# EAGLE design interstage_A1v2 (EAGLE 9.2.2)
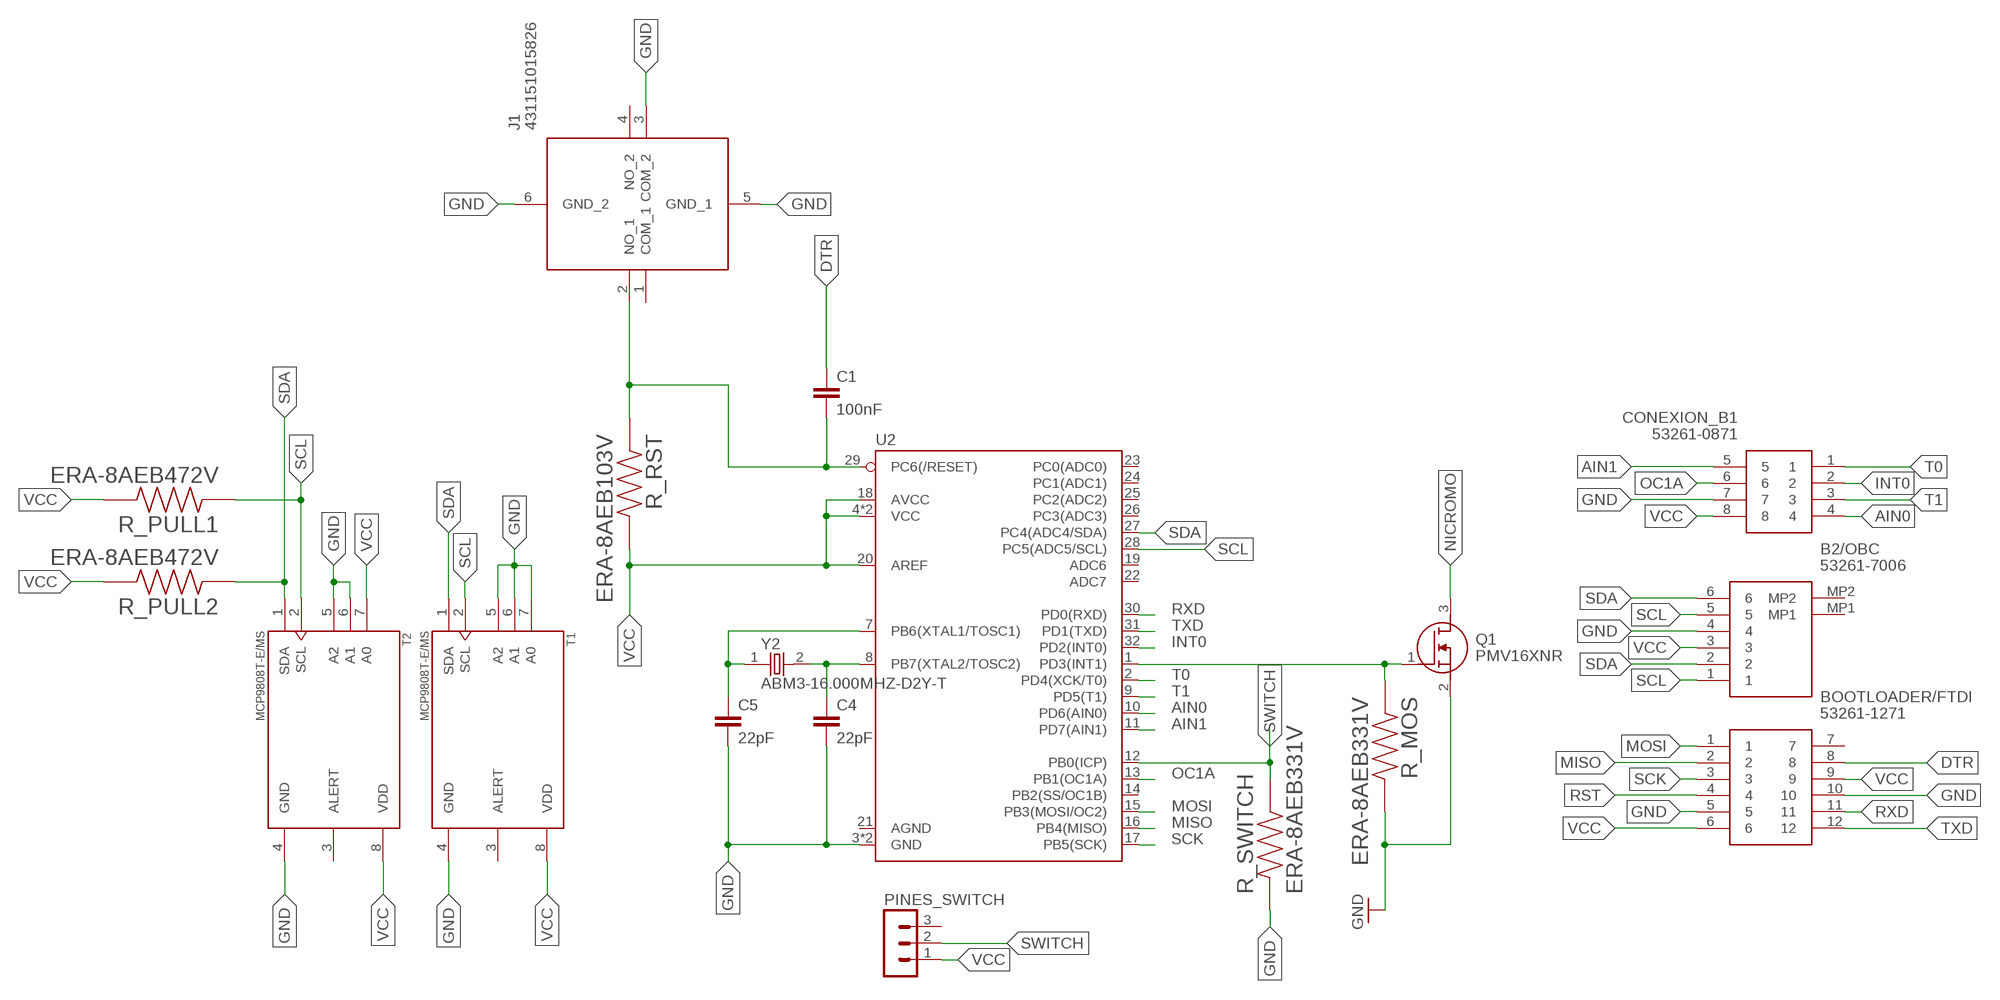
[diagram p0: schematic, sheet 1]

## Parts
B2/OBC  53261-7006  [532617006]
BOOTLOADER/FTDI  53261-1271  [53261-1271]
C1  100nF  C-EUC0805K  [C0805K]
C4  22pF  C-EUC0603K  [C0603K]
C5  22pF  C-EUC0603K  [C0603K]
CONEXION_B1  53261-0871  [53261-0871]
J1  431151015826  [431151015826]
PINES_SWITCH  MA03-1  [MA03-1]
Q1  PMV16XNR  [SOT95P230X110-3N]
R_MOS  ERA-8AEB331V  [RESC3216X70N]
R_PULL1  ERA-8AEB472V  [RESC3216X70N]
R_PULL2  ERA-8AEB472V  [RESC3216X70N]
R_RST  ERA-8AEB103V  [RESC3216X70N]
R_SWITCH  ERA-8AEB331V  [RESC3216X70N]
T1  MCP9808T-E/MS  [SOP65P490X110-8N]
T2  MCP9808T-E/MS  [SOP65P490X110-8N]
U2  ATMEGA328P_TQFP  [TQFP32-08]
Y2  ABM3-16.000MHZ-D2Y-T  [XTAL500X320X130N]

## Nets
AIN0: CONEXION_B1.4 U2.10(PD6(AIN0))
AIN1: CONEXION_B1.5 U2.11(PD7(AIN1))
DTR: BOOTLOADER/FTDI.8 C1.1
GND: B2/OBC.4 BOOTLOADER/FTDI.5 BOOTLOADER/FTDI.10 C4.2 C5.2 CONEXION_B1.7 J1.3(COM_2) J1.5(GND_1) J1.6(GND_2) Q1.2(S) R_MOS.2 R_SWITCH.1 T1.4(GND) T1.5(A2) T1.6(A1) T1.7(A0) T2.4(GND) T2.5(A2) T2.6(A1) U2.3(GND) U2.5(GND)
INT0: CONEXION_B1.2 U2.32(PD2(INT0))
INT1: Q1.1(G) R_MOS.1 U2.1(PD3(INT1))
MISO: BOOTLOADER/FTDI.2 U2.16(PB4(MISO))
MOSI: BOOTLOADER/FTDI.1 U2.15(PB3(MOSI/OC2))
N$1: C5.1 U2.7(PB6(XTAL1/TOSC1)) Y2.1
N$2: C4.1 U2.8(PB7(XTAL2/TOSC2)) Y2.2
NICROMO: Q1.3(D)
OC1A: CONEXION_B1.6 U2.13(PB1(OC1A))
RST: BOOTLOADER/FTDI.4 C1.2 J1.2(NO_1) R_RST.1 U2.29(PC6(/RESET))
RXD: BOOTLOADER/FTDI.11 U2.30(PD0(RXD))
SCK: BOOTLOADER/FTDI.3 U2.17(PB5(SCK))
SCL: B2/OBC.1 B2/OBC.5 R_PULL1.1 T1.2(SCL) T2.2(SCL) U2.28(PC5(ADC5/SCL))
SDA: B2/OBC.2 B2/OBC.6 R_PULL2.1 T1.1(SDA) T2.1(SDA) U2.27(PC4(ADC4/SDA))
SWITCH: PINES_SWITCH.2 R_SWITCH.2 U2.12(PB0(ICP))
T0: CONEXION_B1.1 U2.2(PD4(XCK/T0))
T1: CONEXION_B1.3 U2.9(PD5(T1))
TXD: BOOTLOADER/FTDI.12 U2.31(PD1(TXD))
VCC: B2/OBC.3 BOOTLOADER/FTDI.6 BOOTLOADER/FTDI.9 CONEXION_B1.8 PINES_SWITCH.1 R_PULL1.2 R_PULL2.2 R_RST.2 T1.8(VDD) T2.7(A0) T2.8(VDD) U2.4(VCC) U2.6(VCC) U2.18(AVCC) U2.20(AREF)
Unconnected: B2/OBC.MP1 B2/OBC.MP2 BOOTLOADER/FTDI.7 J1.1(COM_1) J1.4(NO_2) PINES_SWITCH.3 T1.3(ALERT) T2.3(ALERT) U2.14(PB2(SS/OC1B)) U2.19(ADC6) U2.21(AGND) U2.22(ADC7) U2.23(PC0(ADC0)) U2.24(PC1(ADC1)) U2.25(PC2(ADC2)) U2.26(PC3(ADC3))

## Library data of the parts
B2/OBC = SamacSys_Parts:53261-7006: 1.25mm Pitch, PicoBlade PCB Header, Single Row, Right-Angle, Surface Mount, Gold (Au) Plating, Friction Lock, Circuits, Tape and Reel Source: Datasheet; DESCRIPTION: 1.25mm Pitch, PicoBlade PCB Header, Single Row, Right-Angle, Surface Mount, Gold (Au) Plating, Friction Lock, Circuits, Tape and Reel; HEIGHT: 3.6mm; MANUFACTURER_NAME: Molex; MANUFACTURER_PART_NUMBER: 53261-7006; MOUSER_PART_NUMBER: 538-53261-7006; MOUSER_PRICE-STOCK: https://www.mouser.co.uk/ProductDetail/Molex/53261-7006?qs=0lSvoLzn4L%2FSBef0BTU2GA%3D%3D
BOOTLOADER/FTDI = SamacSys_Parts:53261-1271: Molex PICOBLADE Series, Series Number 53261, 1.25mm Pitch 12 Way 1 Row Right Angle PCB Header, Solder Termination, 1A Source: Datasheet; DESCRIPTION: Molex PICOBLADE Series, Series Number 53261, 1.25mm Pitch 12 Way 1 Row Right Angle PCB Header, Solder Termination, 1A; HEIGHT: mm; MANUFACTURER_NAME: Molex; MANUFACTURER_PART_NUMBER: 53261-1271; MOUSER_PART_NUMBER: 538-53261-1271; MOUSER_PRICE-STOCK: https://www.mouser.co.uk/ProductDetail/Molex/53261-1271?qs=%252B72YyncTwW8ciqCjtXK7Ww%3D%3D
C1 C4 C5 = rcl:C-EU: CAPACITOR, European symbol; SPICEPREFIX: C
CONEXION_B1 = SamacSys_Parts:53261-0871: Molex PICOBLADE Series, Series Number 53261, 1.25mm Pitch, 8 Way 1 Row Shrouded Right Angle PCB Header, Surface Mount Source: Datasheet; DESCRIPTION: Molex PICOBLADE Series, Series Number 53261, 1.25mm Pitch, 8 Way 1 Row Shrouded Right Angle PCB Header, Surface Mount; HEIGHT: mm; MANUFACTURER_NAME: Molex; MANUFACTURER_PART_NUMBER: 53261-0871; MOUSER_PART_NUMBER: 538-53261-0871; MOUSER_PRICE-STOCK: https://www.mouser.co.uk/ProductDetail/Molex/53261-0871?qs=%252B72YyncTwW%252BggfdCJ7Netw%3D%3D
J1 = SamacSys_Parts:431151015826: White Tactile Tactile Switch, NO 20 mA 0.3mm Surface Mount Source: Datasheet; DESCRIPTION: White Tactile Tactile Switch, NO 20 mA 0.3mm Surface Mount; HEIGHT: 1.6mm; MANUFACTURER_NAME: Wurth Elektronik; MANUFACTURER_PART_NUMBER: 431151015826; MOUSER_PART_NUMBER: 710-431151015826; MOUSER_PRICE-STOCK: https://www.mouser.co.uk/ProductDetail/Wurth-Elektronik/431151015826?qs=wr8lucFkNMWt0fEnpc%252BesA%3D%3D
PINES_SWITCH = con-lstb:MA03-1: PIN HEADER; OC_FARNELL: unknown; OC_NEWARK: unknown
Q1 = SamacSys_Parts:PMV16XNR: Nexperia PMV16XNR N-channel MOSFET, 8.6 A, 20 V PMV16XN, 3-Pin SOT-23 Source: Datasheet; DESCRIPTION: Nexperia PMV16XNR N-channel MOSFET, 8.6 A, 20 V PMV16XN, 3-Pin SOT-23; HEIGHT: 1.1mm; MANUFACTURER_NAME: Nexperia; MANUFACTURER_PART_NUMBER: PMV16XNR; MOUSER_PART_NUMBER: 771-PMV16XNR; MOUSER_PRICE-STOCK: https://www.mouser.com/Search/Refine.aspx?Keyword=771-PMV16XNR
R_MOS R_SWITCH = resistor_330_smd:ERA-8AEB331V; DESCRIPTION: 330 Ohms ±0.1% 0.25W, 1/4W Chip Resistor 1206 (3216 Metric) Automotive AEC-Q200 Thin Film; DIGI-KEY_PART_NUMBER: P330BCCT-ND; MF: Panasonic Electronic; MP: ERA-8AEB331V; PACKAGE: 3216 Panasonic Electronic Components
R_PULL1 R_PULL2 = resistor_4700_smd:ERA-8AEB472V; DESCRIPTION: RES SMD 4.7K OHM 0.1% 1/4W 1206; DIGI-KEY_PART_NUMBER: P4.7KBCCT-ND; DIGIKEY-PURCHASE-URL: https://snapeda.com/shop?store=DigiKey&id=3718815; MF: Panasonic; MP: ERA-8AEB472V; PACKAGE: 3216 Panasonic Electronic Components
R_RST = resistor_10000_smd:ERA-8AEB103V; DESCRIPTION: 10 kOhms ±0.1% 0.25W, 1/4W Chip Resistor 1206 (3216 Metric) Automotive AEC-Q200 Thin Film; DIGI-KEY_PART_NUMBER: P10KBCCT-ND; DIGIKEY-PURCHASE-URL: https://snapeda.com/shop?store=DigiKey&id=3229630; MF: Panasonic Electronic Components; MP: ERA-8AEB103V; PACKAGE: 3216 Panasonic Electronic Components
T1 T2 = sensorSPEL:MCP9808T-E/MS: Board Mount Temperature Sensors Silicon temp sensor with I2C interface; DESCRIPTION: Temperature Sensor Digital, Local -40°C ~ 125°C 10 b 8-MSOP; DIGI-KEY_PART_NUMBER: MCP9808T-E/MSCT-ND; MF: Microchip; MP: MCP9808T-E/MS; PACKAGE: MSOP-8 Microchip
U2 = SparkFun-IC-Microcontroller:ATMEGA328P_TQFP: Popular 328P in QFP Storefront component: ATmega328 - TQFP (COM-13448) Datasheet SparkFun Products SparkFun RedBoard - Programmed with Arduino (DEV-12757) Arduino Pro Mini 328 - 5V/16MHz (DEV-11113) Arduino Pro Mini 328 - 3.3V/8MHz (DEV-11114) SparkFun OpenLog (DEV-13712) SparkFun MicroView - OLED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; PROD_ID: IC-09069
Y2 = ABM3-16.000MHZ-D2Y-T:ABM3-16.000MHZ-D2Y-T: Crystals 12MHz 18pF 30ppm -40C +85C; DESCRIPTION: 16MHz ±20ppm Crystal 18pF 40 Ohms 2-SMD, No Lead; DIGI-KEY_PART_NUMBER: 535-10638-1-ND; DIGIKEY-PURCHASE-URL: https://snapeda.com/shop?store=DigiKey&id=55267; MF: Abracon; MP: ABM3-16.000MHZ-D2Y-T; PACKAGE: SMD-2 Abracon

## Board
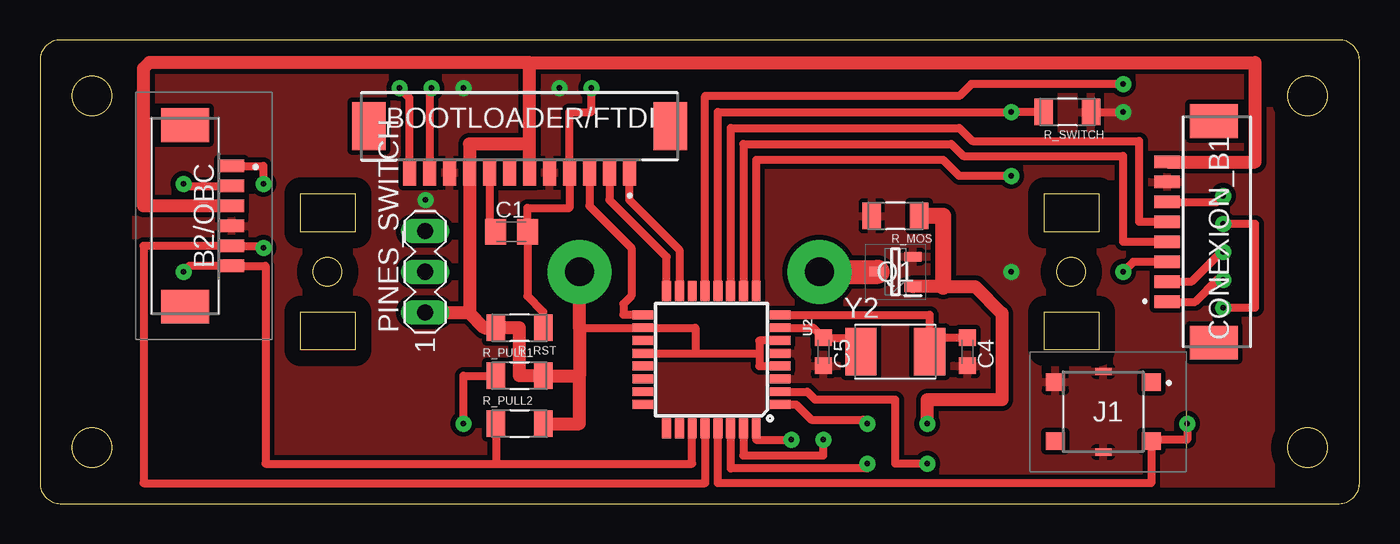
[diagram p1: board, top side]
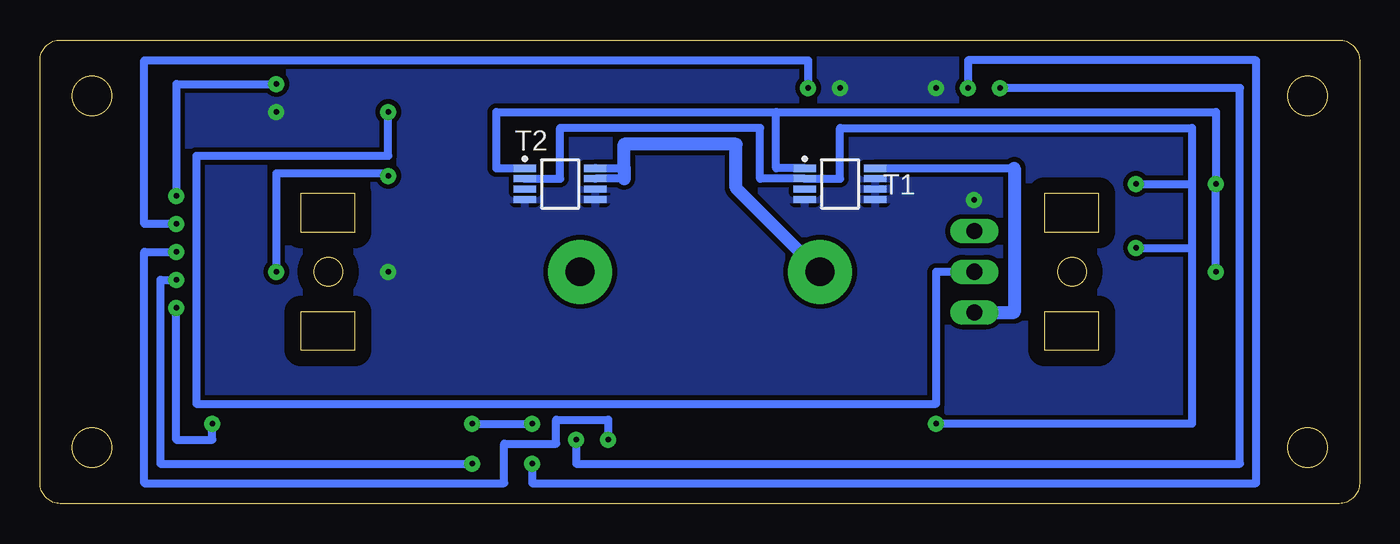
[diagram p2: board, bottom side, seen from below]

Size 82.5 x 29 mm. Coordinates in mm from the lower left corner, seen from the top.
Outline: 16.3,17 16.3,19.4 19.7,19.4 19.7,17 16.3,17
Outline: 62.8,9.6 62.8,12 66.2,12 66.2,9.6 62.8,9.6
Outline: 16.3,9.6 16.3,12 19.7,12 19.7,9.6 16.3,9.6
Outline: 62.8,17 62.8,19.4 66.2,19.4 66.2,17 62.8,17
Outline: 0,1.27 arc90 1.27,0 81.23,0 arc90 82.5,1.27 82.5,27.73 arc90 81.23,29 1.27,29 arc90 0,27.73 0,1.27
Outline: circle at 3.25,25.5 radius 1.25
Outline: circle at 79.25,3.5 radius 1.25
Outline: circle at 79.25,25.5 radius 1.25
Outline: circle at 3.25,3.5 radius 1.25
Outline: circle at 17.98,14.5 radius 0.9
Outline: circle at 64.48,14.5 radius 0.9
Copper layers (1*16): Top 0.035mm / dielectric 1.5mm / Bottom 0.035mm
Design rules "default *": minimum track width 6mil, minimum drill 0.35mm, track to track 0.3mm, track to pad 6mil, pad to pad 6mil, via to via 6mil, smd to smd 6mil, copper to edge 40mil, drill to drill 6mil, minimum pad ring 10mil, minimum via ring 8mil, stop-mask expansion 4mil, vias tented up to drill 0mil, thermal gap 10mil

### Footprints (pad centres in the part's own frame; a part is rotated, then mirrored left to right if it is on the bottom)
532617006 = smd 0.8 x 1.6: 1 3.125,-2.5; 2 1.875,-2.5; 3 0.625,-2.5; 4 -0.625,-2.5; 5 -1.875,-2.5; 6 -3.125,-2.5 | smd 2.1 x 3: MP1 5.675,0.4; MP2 -5.675,0.4
53261-1271 = smd 0.8 x 1.6: 1 -6.875,0.8; 2 -5.625,0.8; 3 -4.375,0.8; 4 -3.125,0.8; 5 -1.875,0.8; 6 -0.625,0.8; 7 0.625,0.8; 8 1.875,0.8; 9 3.125,0.8; 10 4.375,0.8; 11 5.625,0.8; 12 6.875,0.8 | smd 2.1 x 3: 13 -9.425,-2.1; 14 9.425,-2.1
C0805K = smd 1.3 x 1.6: 1 -1,0; 2 1,0
C0603K = smd 1.05 x 1.08: 1 -0.875,0; 2 0.875,0
53261-0871 = smd 0.8 x 1.6: 1 -4.375,1.004; 2 -3.125,1.004; 3 -1.875,1.004; 4 -0.625,1.004; 5 0.625,1.004; 6 1.875,1.004; 7 3.125,1.004; 8 4.375,1.004 | smd 2.1 x 3: 9 6.925,-1.896; 10 -6.925,-1.896
431151015826 = smd 1.2 x 1.1: 1 -3,-1.85; 2 -3,1.85; 3 3,-1.85; 4 3,1.85 | smd 1 x 0.45: 5 0,-2.525; 6 0,2.525
MA03-1 = drill 1.016 long: 1 -2.54,0; 2 0,0; 3 2.54,0
SOT95P230X110-3N = smd 1.05 x 0.6: 1 -1.1,0.95; 2 -1.1,-0.95; 3 1.1,0
RESC3216X70N = smd 1.16 x 1.68: 1 -1.475,0; 2 1.475,0
SOP65P490X110-8N = smd 1.4 x 0.45: 1 -2.2,0.975; 2 -2.2,0.325; 3 -2.2,-0.325; 4 -2.2,-0.975; 5 2.2,-0.975; 6 2.2,-0.325; 7 2.2,0.325; 8 2.2,0.975
TQFP32-08 = smd 1.27 x 0.559: 1 -4.293,2.8; 2 -4.293,2; 3 -4.293,1.2; 4 -4.293,0.4; 5 -4.293,-0.4; 6 -4.293,-1.2; 7 -4.293,-2; 8 -4.293,-2.8; 17 4.293,-2.8; 18 4.293,-2; 19 4.293,-1.2; 20 4.293,-0.4; 21 4.293,0.4; 22 4.293,1.2; 23 4.293,2; 24 4.293,2.8 | smd 0.559 x 1.27: 9 -2.8,-4.293; 10 -2,-4.293; 11 -1.2,-4.293; 12 -0.4,-4.293; 13 0.4,-4.293; 14 1.2,-4.293; 15 2,-4.293; 16 2.8,-4.293; 25 2.8,4.293; 26 2,4.293; 27 1.2,4.293; 28 0.4,4.293; 29 -0.4,4.293; 30 -1.2,4.293; 31 -2,4.293; 32 -2.8,4.293
XTAL500X320X130N = smd 1.95 x 2.95: 1 -2.15,0; 2 2.15,0

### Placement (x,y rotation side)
B2/OBC  9.48,18 90 top
BOOTLOADER/FTDI  29.98,21.5 180 top
C1  29.48,17 0 top
C4  57.98,9.5 270 top
C5  48.98,9.5 270 top
CONEXION_B1  71.48,17 90 top
J1  66.48,5.75 180 top
PINES_SWITCH  24.08,14.5 90 top
Q1  53.48,14.5 180 top
R_MOS  53.48,18 180 top
R_PULL1  29.98,8 0 top
R_PULL2  29.98,5 0 top
R_RST  29.98,11 180 top
R_SWITCH  64.23,24.5 180 top
T1  32.48,20 0 bottom
T2  49.98,20 0 bottom
U2  41.98,9 180 top
Y2  53.48,9.5 0 top

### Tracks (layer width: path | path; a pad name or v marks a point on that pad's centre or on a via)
AIN0
  Top 0.5: U2.10 43.98,22.5 56.98,22.5 57.73,21.75 67.73,21.75 67.73,16.38 CONEXION_B1.4
AIN1
  Top 0.5: U2.11 43.18,23.5 57.48,23.5 58.3,22.68 68.73,22.68 68.73,17.62 CONEXION_B1.5
DTR
  Top 0.5: BOOTLOADER/FTDI.8 28.11,17.38 C1.1
GND  (via drill 0.35 pad 1)
  Top 0.5: R_SWITCH.1 v67.73,24.5
  other vias: 26.48,26 32.48,26 60.73,14.5 24.11,19
  pour Top (isolate 0.25): 5.98,28.5 5.98,0.5 76.98,0.5 76.98,28.5
  pour Bottom (isolate 0.25): 76.98,0.5 76.98,28.5 5.98,28.5 5.98,0.5
INT0  (via drill 0.35 pad 1)
  Top 0.5: U2.32 44.78,4 v46.98,4 | CONEXION_B1.2 71.98,13.88 73.85,15.75 v73.98,15.75
  Bottom 0.5: v73.98,15.75 75.98,15.75 75.98,1.27 53.48,1.27 53.48,3.75 50.23,3.75 50.23,5.25 46.98,5.25 v46.98,4
INT1  (via drill 0.35 pad 1)
  Top 0.5: U2.1 47.28,6.2 48.23,5.25 51.48,5.25 v51.73,5 | 54.61,13.58 Q1.1
  Top 0.8: v55.48,5 55.48,6.5 60.15,6.5 60.15,11.9 58.48,13.58 56.48,13.58 54.61,13.58
  Top 1: 56.48,13.58 56.48,18 R_MOS.1
  Bottom 0.5: v55.48,5 v51.73,5
MISO
  Top 0.5: U2.16 39.18,15.43 35.6,19 BOOTLOADER/FTDI.2
MOSI
  Top 0.5: U2.15 39.98,15.88 36.85,19 BOOTLOADER/FTDI.1
N$1
  Top 0.5: U2.7 48.35,11 C5.1 50.45,10.38 Y2.1
N$2
  Top 0.5: U2.8 55.63,11.8 Y2.2 56.5,10.38 C4.1
NICROMO  (via drill 1.8 pad 4)
  Top 1.5: v48.73,14.5 Q1.3
OC1A  (via drill 0.35 pad 1)
  Top 0.5: U2.13 41.58,25.5 57.48,25.5 58.23,26.25 v67.73,26.25 | v73.98,19.25 73.61,18.88 CONEXION_B1.6
  Bottom 0.5: v73.98,19.25 73.98,26.25 v67.73,26.25
RST  (via drill 0.35 pad 1)
  Top 0.5: v73.98,12.25 75.98,12.25 75.98,17.5 v73.98,17.5 | v34.48,26 34.48,24.5 33.1,24.5 BOOTLOADER/FTDI.4 33.1,18.5 30.48,18.5 C1.2 30.48,12.97 31.46,12 R_RST.1 | U2.29 42.38,1.27 69.48,1.27 J1.2 69.48,4 71.73,4 v71.73,5
  Bottom 0.5: v73.98,17.5 75.98,17.5 75.98,27.73 34.48,27.73 v34.48,26 | v73.98,12.25 73.98,4 71.73,4 v71.73,5
RXD  (via drill 0.35 pad 1)
  Top 0.5: v51.73,2.5 51.73,2.2 43.18,2.2 U2.30 | v24.48,26 24.36,25.88 BOOTLOADER/FTDI.11
  Bottom 0.5: v51.73,2.5 51.73,1.27 6.48,1.27 6.48,27.73 24.48,27.73 v24.48,26
SCK
  Top 0.5: U2.17 36.48,11.8 36.48,12.5 36.98,13 36.98,16 34.35,18.62 BOOTLOADER/FTDI.3
SCL  (via drill 0.35 pad 1)
  Top 0.5: U2.28 41.58,1.27 6.48,1.27 6.48,16.12 B2/OBC.5 13.98,16.12 v13.98,16 | v13.98,20 13.98,21.12 B2/OBC.1 | R_PULL1.1 26.48,8 v26.48,5
  Bottom 0.5: T2.2 49.98,20.32 49.98,23.5 37.48,23.5 37.48,20.32 T1.2 32.48,20.32 32.48,23.5 10.48,23.5 10.48,20 | v13.98,20 10.48,20 | 10.48,20 10.48,16 | 10.48,16 10.48,5 v26.48,5 | v13.98,16 10.48,16
SDA  (via drill 0.35 pad 1)
  Top 0.5: U2.27 40.78,2.5 28.48,2.5 | 28.48,2.5 14.11,2.5 14.11,14.88 B2/OBC.6 9.36,14.88 v8.98,14.5 | v8.98,20 9.11,19.88 B2/OBC.2 | R_PULL2.1 28.5,2.52 28.48,2.5
  Bottom 0.5: v8.98,14.5 v8.98,20 8.98,24.5 36.48,24.5 | T2.1 53.98,20.98 53.98,24.5 36.48,24.5 | T1.1 36.48,20.98 36.48,24.5
SWITCH  (via drill 0.35 pad 1)
  Top 0.5: U2.12 42.38,24.5 v60.73,24.5 R_SWITCH.2
  Bottom 0.5: v60.73,24.5 60.73,21.75 72.73,21.75 72.73,6.25 26.48,6.25 26.48,14.5 PINES_SWITCH.2
T0  (via drill 0.35 pad 1)
  Top 0.5: U2.2 47.98,7 48.48,6.5 53.48,6.5 53.48,2.5 v55.48,2.5 | v73.98,14 73.6,14 72.23,12.62 CONEXION_B1.1
  Bottom 0.5: v73.98,14 74.98,14 74.98,2.5 v55.48,2.5
T1  (via drill 0.35 pad 1)
  Top 0.5: U2.9 44.78,21.5 56.48,21.5 57.48,20.5 v60.73,20.5 | CONEXION_B1.3 68.36,15.12 v67.73,14.5
  Bottom 0.5: v60.73,20.5 60.73,20.67 67.73,20.67 v67.73,14.5
TXD  (via drill 0.35 pad 1)
  Top 0.5: v48.98,4 48.98,3 43.98,3 U2.31 | v22.48,26 23.11,25.38 BOOTLOADER/FTDI.12
  Bottom 0.5: v48.98,4 48.98,2.5 7.48,2.5 7.48,26 v22.48,26
VCC  (via drill 1.8 pad 4)
  Top 0.5: U2.4 44.98,8.6 44.98,9.4 | U2.6 44.98,10.2 44.98,9.4 | U2.20 40.98,9.4 | 40.98,9.4 44.98,9.4 | 40.98,9.4 40.98,11 U2.18 33.73,11 | 26.86,21.5 BOOTLOADER/FTDI.9 | 26.82,11.96 26.86,12
  Top 0.8: CONEXION_B1.8 75.98,21.38 75.98,27.58 30.61,27.58 | v33.73,14.5 33.73,11 33.73,8 | BOOTLOADER/FTDI.9 26.86,12 | B2/OBC.3 6.48,18.62 6.48,27.23 6.83,27.58 30.61,27.58 | PINES_SWITCH.1 26.82,11.96 27.78,11 R_RST.2 29.98,11 29.98,8 R_PULL1.2 33.73,8 | R_PULL2.2 33.73,5 33.73,8 | 30.61,22.5 26.86,22.5 26.86,21.5 | BOOTLOADER/FTDI.6 30.61,22.5 | 30.61,22.5 30.61,27.58
  Bottom 0.5: T1.8 21.58,20.98 | T2.8 47.78,21 45.98,21 | 45.98,20.32 T2.7
  Bottom 0.8: 21.58,20.98 21.58,11.96 PINES_SWITCH.1 | 45.98,20.32 45.98,21 45.98,22.48 38.98,22.48 38.98,19.75 v33.73,14.5

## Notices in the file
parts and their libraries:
SparkFun-IC-Microcontroller: Licensing: Creative Commons ShareAlike 4.0 International - https://creativecommons.org/licenses/by-sa/4.0
